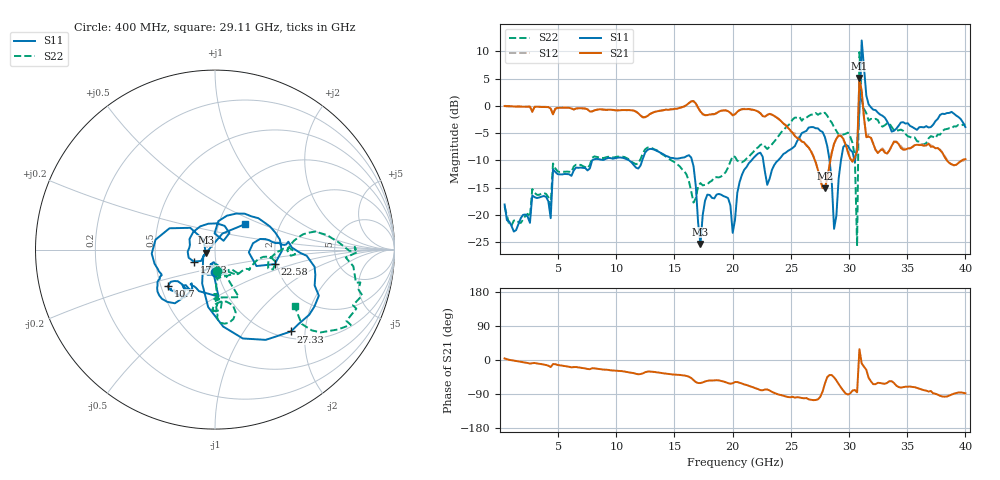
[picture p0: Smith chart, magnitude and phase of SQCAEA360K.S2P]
! Network Analyzer HP8722ES.07.66: Jul 25, 2000 Serial No. US39175408
! 27 Oct 2004  10:40:29
! Frequency  S11  S21  S12  S22
# HZ  S  DB R  50
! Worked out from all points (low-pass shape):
!   201 points, 400 MHz to 40 GHz, reference 50 ohm
!   highest |S21| = 5.10 dB at 30.89 GHz (marker M1); lowest = -15.1 dB at 27.92 GHz (marker M2)
!   |S21| within 3 dB of the highest: 30.85 GHz to 31.11 GHz (265.8 MHz wide, 0.858 % of centre)
!   lowest |S11| = -25.3 dB at 17.23 GHz (marker M3), VSWR 1.11, Z = 45.1 - j1.48 ohm
!   |S11| at or under -10 dB: start of sweep to 7.921 GHz; 16.5 GHz to 21.61 GHz (5.111 GHz wide, 26.8 % of centre); 22.62 GHz to 23.9 GHz (1.273 GHz wide, 5.47 % of centre)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
!   |S22| runs from -25.7 to 9.8 dB; largest |S21 - S12| = 0.51
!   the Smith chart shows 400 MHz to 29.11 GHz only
!   S11 on the Smith chart (normalised r, x): 400 MHz: 0.97, -0.25; 10.7 GHz: 0.55, -0.25; 17.63 GHz: 0.78, -0.11; 22.58 GHz: 1.95, -0.36; 27.33 GHz: 1.14, -1.69; 29.11 GHz: 1.33, +0.39
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4e8  -18.07 -90.5  -0.04 4.1  0.03 4.9  -18.44 -85.0
7.132e9  -11.37 -131.0  -0.45 -21.2  -0.50 -21.7  -11.04 -91.3
1.0696e10  -9.61 -142.2  -0.77 -30.5  -0.77 -31.0  -9.37 -92.4
1.3666e10  -8.45 -148.0  -0.94 -33.4  -0.90 -33.8  -8.48 -88.2
1.6438e10  -9.47 170.5  0.82 -47.6  0.83 -48.6  -15.65 -85.1
1.723e10  -25.30 -162.4  -1.04 -60.9  -1.07 -61.4  -14.15 -47.9
1.7626e10  -17.37 -150.5  -1.71 -56.7  -1.71 -57.2  -14.47 -43.7
2.02e10  -20.89 91.6  -1.53 -58.0  -1.55 -58.5  -9.34 -18.9
2.2576e10  -9.31 -13.7  -1.88 -79.9  -1.79 -80.7  -6.99 -3.4
2.6932e10  -3.90 -34.7  -9.27 -106.0  -9.15 -106.7  -1.62 -15.6
2.7328e10  -4.12 -47.1  -11.74 -103.8  -11.85 -102.8  -1.63 -21.9
2.7922e10  -5.70 -72.6  -15.13 -62.7  -15.09 -61.9  -1.26 -29.0
2.8714e10  -22.52 -151.2  -6.97 -45.8  -6.88 -47.4  -3.93 -40.6
2.911e10  -13.29 40.5  -5.47 -63.6  -5.30 -64.6  -5.28 -35.3
3.0496e10  -10.24 6.5  -9.45 -79.2  -9.31 -79.6  -9.24 -40.4
3.0694e10  -7.50 17.4  -8.28 -85.3  -8.18 -85.6  -25.71 1.9
3.0892e10  -1.08 24.0  5.10 28.4  2.19 28.4  9.84 -83.5
3.109e10  11.98 -6.9  2.67 -9.1  2.44 -10.3  1.02 -58.7
3.1288e10  7.00 -42.5  -2.18 -17.8  -2.29 -18.5  -0.55 -37.6
3.1486e10  1.87 -45.4  -5.75 -25.9  -5.57 -28.4  -1.35 -26.7
3.3466e10  -3.62 -76.1  -8.16 -56.0  -8.23 -56.5  -3.21 -26.3
4e10  -3.89 -81.1  -9.77 -87.9  -9.84 -89.6  -3.40 -37.6
